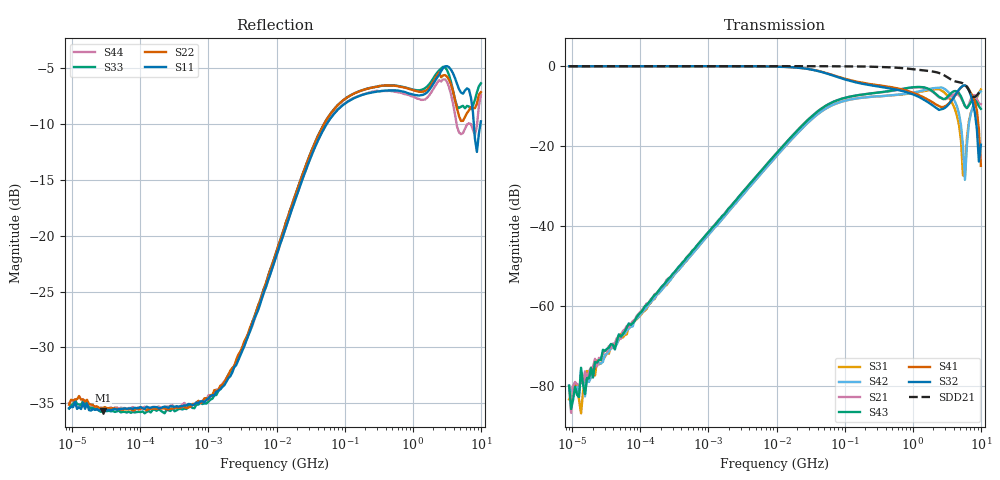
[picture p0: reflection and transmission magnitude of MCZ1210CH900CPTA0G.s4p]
! S-Parameter Data Generated by TDK Corporation
! Copyright(C) 2024 TDK Corporation.
! All Rights Reserved.
! TDK P/N: MCZ1210CH900CPTA0G (Signal Line Common Mode Choke/Filter)
! Property: |Zc|=90ohm at 100MHz
! Size(LxWxT): 1.25x1x0.5mm
! Model Type: s2p (Touchstone File Format Version 1.0)
! Frequency: DC=Yes Start=0.009MHz Stop=10000MHz 209points Log-sweep
! Model Generated on May 28, 2024
! Terms and conditions regarding TDK Simulation Models:
! 1)This simulation model is being provided solely for informational
!  purposes. Please refer to the specifications of the products in
!  terms of detailed characteristics of such products.
! 2)In no event shall TDK Corporation of any of its subsidiaries be
!  liable for any loss or damage arising, directly or indirectly,
!  from any information contained in this simulation model, including,
!  but not limited to loss or damages arising from any inaccuracies,
!  omissions or errors in connection with such information.
! 3)Any and all copyrights on this simulation model are owned by
!  TDK Corporation.  Duplication or redistribution of this simulation
!  model without prior written permission from TDK Corporation
!  is prohibited.
! 4)This simulation model is subject to any modification or change
!  without any prior notice.
! 5)Neither TDK Corporation nor any of its subsidiaries shall make any
!  warranty, express or implied, including but not limited to the
!  correctness, implied warranties of merchantability and fitness for
!  a particular purpose with respect to this simulation models.
! 6)The use of this simulation model shall be deemed to have consented
!  to the terms and conditions hereof.
! Port Assignments:
!  1 ---@@@--- 4
!  2 ---@@@--- 3
! Applicable Conditions:
!  Temperature = 25 degC
!  DC Bias Current = 0 A
!  Small Signal Operation
# Hz S MA R 50
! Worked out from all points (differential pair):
!   208 points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, 9 kHz to 10 GHz, reference 50 ohm
!   strongest paths, dB at 9 kHz, 297.2 kHz, 9.811 MHz, 323.9 MHz, 10 GHz:
!     S32: -0.2, -0.1, -0.2, -5.3, -19.8
!     S41: -0.2, -0.2, -0.3, -4.9, -25.0
!     S43: -80.0, -52.1, -22.0, -6.7, -10.8
!     S21: -80.0, -52.2, -22.0, -6.7, -9.6
!     S42: -80.0, -52.7, -22.8, -7.7, -6.5
!     S31: -83.4, -52.8, -22.7, -7.7, -6.0
!   taken as a pair (ports 2,1 in; 3,4 out), SDD21 dB: -0.2, -0.1, -0.2, -0.3, -6.0
!   lowest |S11| = -35.7 dB at 28.23 kHz (marker M1), VSWR 1.03, Z = 51.7 + j0.0279 ohm
!   |S11| at or under -10 dB: start of sweep to 54.58 MHz; 7.882 GHz to 9.858 GHz (1.976 GHz wide, 22.3 % of centre)
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9000  0.0169 3.4  0.0001155 86.8  0.0001427 -97.9  0.9832 -0.1
      0.0001001 41.1  0.01751 22.0  0.9826 -0.2  9.067e-05 -139.9
      6.762e-05 -108.0  0.9828 -0.2  0.01684 16.0  4.543e-05 90.0
      0.9822 -0.1  0.0001001 -77.6  0.0001005 104.7  0.01787 7.6
28232.8  0.01647 0.9  0.0002484 88.8  0.0001741 -95.0  0.9832 -0.0
         0.0002508 78.8  0.01697 10.3  0.983 -0.2  0.0002187 -94.6
         0.0002134 -77.4  0.9829 -0.1  0.01658 5.7  0.0002335 92.8
         0.9833 -0.0  0.0001998 -92.2  0.0002823 92.1  0.01686 -0.1
1304751  0.02003 30.5  0.0109 88.7  0.01006 -91.4  0.9821 -0.7
         0.01091 88.6  0.02014 33.4  0.9836 -0.7  0.009952 -91.5
         0.009975 -92.1  0.9822 -0.7  0.01936 32.7  0.01085 88.8
         0.983 -0.6  0.009892 -92.0  0.0107 88.3  0.0205 30.3
4.928127e7  0.2997 45.1  0.3041 48.8  0.2805 -135.2  0.8245 -17.4
            0.3039 48.9  0.3143 45.0  0.8184 -18.2  0.2803 -135.3
            0.2801 -135.2  0.818 -18.3  0.3148 45.3  0.304 48.8
            0.8248 -17.4  0.2803 -135.3  0.3041 48.8  0.3007 45.0
2.786605e9  0.5629 -32.7  0.3819 -9.6  0.4747 27.3  0.304 -179.8
            0.382 -9.7  0.5219 -30.9  0.2889 175.1  0.524 26.5
            0.4748 27.2  0.2889 175.1  0.5703 -28.3  0.3823 -7.2
            0.3042 -179.9  0.5243 26.6  0.3824 -7.3  0.5007 -26.8
5.839122e9  0.4468 -39.7  0.311 -9.7  0.04143 105.1  0.5646 31.4
            0.3112 -9.6  0.3401 -59.8  0.5685 32.0  0.03799 -169.1
            0.04173 103.3  0.5671 32.0  0.372 -46.3  0.312 -15.7
            0.566 31.4  0.03746 -170.3  0.3124 -15.7  0.301 -59.7
1e10  0.3251 -46.7  0.329 0.2  0.5106 25.9  0.0568 -168.0
      0.3297 0.1  0.4391 -68.1  0.1051 94.4  0.4744 16.2
      0.503 26.0  0.1029 93.8  0.481 -47.8  0.2842 7.8
      0.05593 -166.4  0.4742 16.4  0.2884 7.7  0.4256 -38.1
